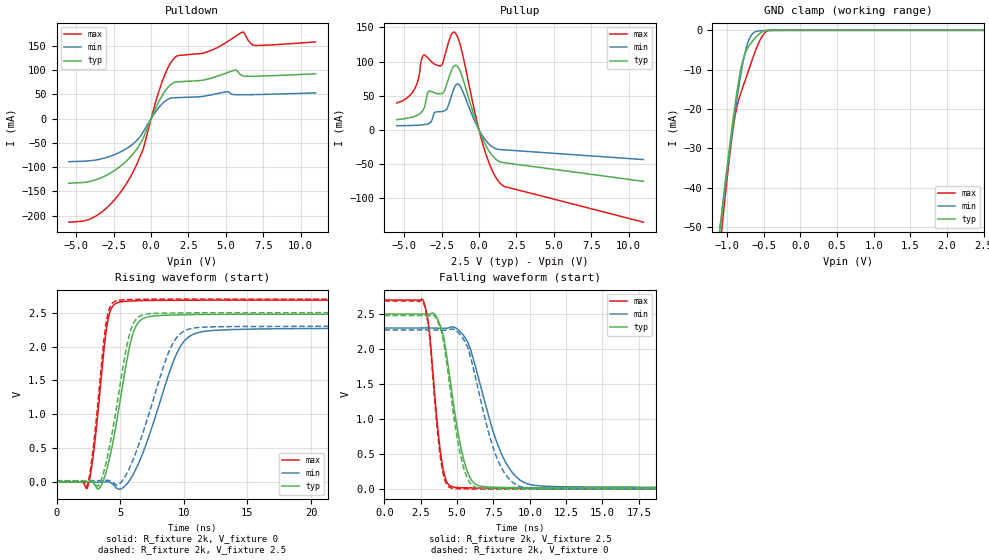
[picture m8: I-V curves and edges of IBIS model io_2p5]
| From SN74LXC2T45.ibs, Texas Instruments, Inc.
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[Model]   io_2p5
Model_type  I/O
Vinl=0.7
Vinh=1.7
Enable   Active-Low
Vref =   0
Rref =   2000
Cref =   15p
Vmeas =   1.25
| variable   typ   min   max
C_comp   6.20pF   5.38pF   7.19pF
| C_pullup   12.65pF   6.38pF   21.50pF
| C_pulldown   9.65pF   6.74pF   15.56pF
| C_tri-state   6.20pF   5.38pF   7.19pF
[Temperature Range]   40   100   -40
| Ambient temperature   25   85   -40
[Voltage range]   2.5   2.3   2.7
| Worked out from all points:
|   slope of the pulldown table from 0 to 0.375 V, typ, clamps not added: 14.3 ohm
|   slope of the pullup table from 0 to 0.375 V, typ, clamps not added: 19.7 ohm
|   GND clamp passes 1 mA (typ) near -0.56 V on its own axis
|   rising waveform, R_fixture 2k, V_fixture 0: 20-80 % time 1.39ns typ, 2.43ns min, 868ps max; typ from 0 V to 2.48 V
|   falling waveform, R_fixture 2k, V_fixture 2.5: 20-80 % time 1.14ns typ, 1.98ns min, 709ps max; typ from 2.5 V to 0.017 V
|   rising waveform, R_fixture 2k, V_fixture 2.5: 20-80 % time 1.37ns typ, 2.35ns min, 853ps max; typ from 0.017 V to 2.5 V
|   falling waveform, R_fixture 2k, V_fixture 0: 20-80 % time 1.06ns typ, 1.72ns min, 683ps max; typ from 2.48 V to 0 V
[GND Clamp]
| LXC8T245_IO_25
|   Voltage   I(typ)   I(min)   I(max)
-5.5V     -897.1mA   -831.9mA   -1.015A
-1.11V    -52.66mA   -52.33mA   -57.72mA
-1.08V    -47.7mA    -47.75mA   -52.14mA
-1.05V    -42.82mA   -43.24mA   -46.67mA
-970mV    -30.27mA   -31.55mA   -32.88mA
-910mV    -21.53mA   -23.26mA   -24.11mA
-825mV    -11.15mA   -12.66mA   -16.7mA
-725mV    -4.734mA   -3.633mA   -11.25mA
-630mV    -2.234mA   -514.4uA   -6.052mA
-515mV    -326.1uA   -90.88uA   -1.362mA
-425mV    -4.501uA   -33.03uA   -11.43uA
2.5V      27.51pA    91.09nA    545.1pA
[Pulldown]
| LXC8T245_IO_25
|   Voltage   I(typ)   I(min)   I(max)
-5.5V     -133.3mA   -88.88mA   -213.8mA
-3.55V    -124.7mA   -84.51mA   -198.3mA
-1.715V   -89.25mA   -63.13mA   -137.4mA
-555mV    -41.71mA   -28.61mA   -64.74mA
300mV     21.24mA    14.01mA    33.98mA
855mV     53.14mA    33.96mA    85.74mA
1.655V    75.71mA    43.25mA    127.8mA
3.765V    81.48mA    47.49mA    138mA
5.655V    100.3mA    49.41mA    170.3mA
6.145V    88.26mA    49.23mA    178.7mA
6.91V     87.46mA    49.58mA    151.3mA
11V       92.57mA    53.16mA    158.4mA
[Pullup]
| LXC8T245_IO_25
|   Voltage   I(typ)   I(min)   I(max)
-5.5V     15.18mA    6.286mA    39.52mA
-4.375V   19.38mA    6.776mA    57.63mA
-3.925V   24.63mA    7.34mA     94.35mA
-3.695V   31.09mA    7.844mA    109.8mA
-3.295V   56.83mA    10.28mA    102.6mA
-2.495V   53.5mA     27.01mA    94.85mA
-2.135V   68.6mA     31.44mA    120.9mA
-1.645V   94.12mA    62.3mA     143.1mA
-1.23V    84.36mA    63.07mA    122.5mA
335mV     -17.24mA   -11.96mA   -26.61mA
1.44V     -46.81mA   -28.58mA   -78.45mA
11V       -75.01mA   -43.22mA   -134.8mA
[Ramp]
| LXC8T245_IO_25
| variable   typ   min   max
dV/dt_r   1.50/0.8E-09   1.35/1.24E-09   1.65/0.63E-10
dV/dt_f   1.50/0.8E-09   1.35/1.7E-09   1.65/0.63E-10
R_load = 2k
[Rising Waveform]
| LXC8T245_IO_25
R_fixture =   2k
C_fixture =   0
L_fixture =   0
V_fixture =   0
V_fixture_min = 0
V_fixture_max = 0
|   Time   V(typ)   V(min)   V(max)
0s        299.6pV    7.204nV    2.034nV
2.46ns    17.85uV    -5.835uV   -65.72mV
2.95ns    -24.7mV    -35.8uV    493mV
3.97ns    202.6mV    6.715mV    2.316V
4.77ns    945.4mV    -96.58mV   2.645V
5.745ns   2.004V     29.08mV    2.671V
6.4ns     2.349V     259.5mV    2.676V
9.37ns    2.467V     1.869V     2.682V
10.9ns    2.472V     2.193V     2.683V
40ns      2.477V     2.27V      2.684V
[Falling Waveform]
| LXC8T245_IO_25
R_fixture =   2k
C_fixture =   0
L_fixture =   0
V_fixture =   2.5
V_fixture_min = 2.3
V_fixture_max = 2.7
|   Time   V(typ)   V(min)   V(max)
0s        2.5V       2.3V       2.7V
2.7ns     2.499V     2.3V       2.677V
3.08ns    2.497V     2.3V       2.27V
3.94ns    2.276V     2.296V     403.2mV
4.64ns    1.38V      2.316V     36.72mV
5.355ns   505.6mV    2.213V     21mV
6.04ns    114.4mV    1.912V     17.82mV
7.985ns   25.21mV    535.9mV    14.24mV
9.845ns   21.9mV     75.58mV    12.99mV
40ns      16.67mV    23.22mV    11.27mV
[Rising Waveform]
| LXC8T245_IO_25
R_fixture =   2k
C_fixture =   0
L_fixture =   0
V_fixture =   2.5
V_fixture_min = 2.3
V_fixture_max = 2.7
|   Time   V(typ)   V(min)   V(max)
0s        16.61mV    22.91mV    11.26mV
2.415ns   16.45mV    22.9mV     -49.97mV
3.285ns   -53.08mV   22.78mV    1.239V
3.89ns    286.3mV    28.18mV    2.337V
4.655ns   1.037V     -38.27mV   2.671V
5.565ns   2.046V     145.5mV    2.692V
6.2ns     2.391V     419.5mV    2.695V
8.85ns    2.494V     1.934V     2.699V
10.31ns   2.497V     2.252V     2.7V
40ns      2.5V       2.3V       2.7V
[Falling Waveform]
| LXC8T245_IO_25
R_fixture =   2k
C_fixture =   0
L_fixture =   0
V_fixture =   0
V_fixture_min = 0
V_fixture_max = 0
|   Time   V(typ)   V(min)   V(max)
0s        2.478V     2.272V     2.685V
2.695ns   2.477V     2.272V     2.662V
3.065ns   2.475V     2.272V     2.253V
3.89ns    2.263V     2.268V     393.9mV
4.545ns   1.392V     2.283V     20.12mV
5.22ns    498.1mV    2.201V     5.542mV
5.885ns   89.91mV    1.915V     3.857mV
7.66ns    3.274mV    487mV      1.965mV
9.385ns   2.437mV    33.38mV    1.267mV
40ns      55.14uV    200uV      6.623uV
